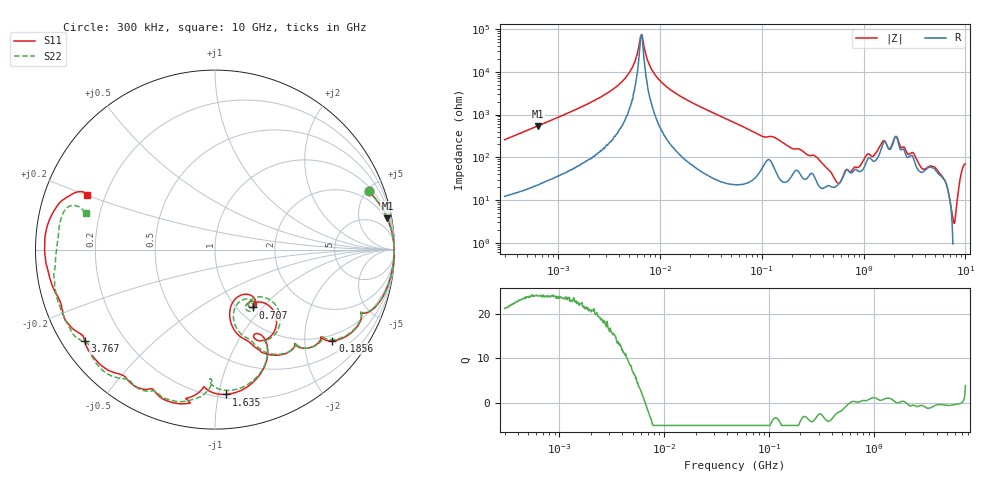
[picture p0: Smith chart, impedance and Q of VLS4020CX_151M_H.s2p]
! S-Parameter Data Generated by TDK Corporation
! Copyright(C) 2024 TDK Corporation.
! All Rights Reserved.
! TDK P/N: VLS4020CX-151M-H (SMD / SMT Inductor (Coil))
! Property: L=150uH at 1MHz
! Size(LxWxT): 4x4x2mm
! Model Type: s2p (Touchstone File Format Version 1.0)
! Frequency: DC=Yes Start=0.3MHz Stop=10000MHz 802points Log-sweep
! Model Generated on May 28, 2024
! Terms and conditions regarding TDK Simulation Models:
! 1)This simulation model is being provided solely for informational
!  purposes. Please refer to the specifications of the products in
!  terms of detailed characteristics of such products.
! 2)In no event shall TDK Corporation of any of its subsidiaries be
!  liable for any loss or damage arising, directly or indirectly,
!  from any information contained in this simulation model, including,
!  but not limited to loss or damages arising from any inaccuracies,
!  omissions or errors in connection with such information.
! 3)Any and all copyrights on this simulation model are owned by
!  TDK Corporation.  Duplication or redistribution of this simulation
!  model without prior written permission from TDK Corporation
!  is prohibited.
! 4)This simulation model is subject to any modification or change
!  without any prior notice.
! 5)Neither TDK Corporation nor any of its subsidiaries shall make any
!  warranty, express or implied, including but not limited to the
!  correctness, implied warranties of merchantability and fitness for
!  a particular purpose with respect to this simulation models.
! 6)The use of this simulation model shall be deemed to have consented
!  to the terms and conditions hereof.
! Port Assignments:
!  1 ---@@@--- 2
! Applicable Conditions:
!  Temperature = 25 degC
!  DC Bias Current = 0 A
!  Small Signal Operation
# Hz S MA R 50
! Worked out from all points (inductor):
!   801 points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, 300 kHz to 10 GHz, reference 50 ohm
!   read as one part in series: L = 135 uH near 318.3 kHz
!   highest Q = 24 at 636.7 kHz (marker M1), where L = 135 uH
!   self-resonance near 6.556 MHz
!   S11 on the Smith chart (normalised r, x): 300 kHz: 1.27, +5.17; 185.6 MHz: 0.83, -2.69; 707 MHz: 1.17, -0.89; 1.635 GHz: 0.23, -1.05; 3.767 GHz: 0.07, -0.31; 10 GHz: 0.13, +0.20
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300000  0.9171 20.7  0.3572 -66.6  0.3572 -66.6  0.9173 20.7
636701  0.9761 10.3  0.1803 -77.3  0.1802 -77.3  0.976 10.3
1713600  0.9949 3.6  0.0656 -83.7  0.06573 -83.7  0.9948 3.6
4487199  0.9984 0.5  0.01487 -83.6  0.01488 -83.5  0.9983 0.5
5416338  0.9986 0.1  0.007638 -80.1  0.007654 -79.6  0.9987 0.1
6556275  0.9987 -0.4  0.001397 -14.9  0.00132 -12.1  0.9987 -0.4
7771787  0.9987 -0.9  0.00614 77.4  0.006137 77.1  0.9988 -0.8
9671944  0.9985 -1.5  0.01459 83.5  0.01462 83.5  0.9987 -1.5
5.477226e7  0.9828 -12.3  0.1533 75.7  0.1534 75.7  0.9827 -12.2
1.855783e8  0.8285 -37.9  0.441 43.4  0.4411 43.4  0.8312 -37.1
3.126428e8  0.691 -49.9  0.5286 21.1  0.5287 21.1  0.6903 -49.3
5.225392e8  0.4301 -77.5  0.7491 -7.9  0.7493 -7.9  0.4364 -75.1
7.069847e8  0.3847 -56.9  0.6277 -32.2  0.6278 -32.2  0.3959 -60.3
9.789263e8  0.4268 -46.2  0.5948 -64.1  0.5949 -64.2  0.3845 -43.9
1.371335e9  0.6406 -62.7  0.3677 -94.6  0.3679 -94.6  0.6674 -64.3
1.635219e9  0.8091 -85.6  0.1862 -83.5  0.1864 -83.5  0.7835 -86.8
1.767019e9  0.7729 -94.0  0.2329 -82.6  0.233 -82.7  0.7231 -92.4
2.112126e9  0.8836 -104.2  0.1123 -80.9  0.1124 -80.9  0.8677 -102.4
3.766866e9  0.8875 -145.0  0.162 -85.5  0.1619 -85.7  0.8922 -141.6
5.849356e9  0.9105 -160.4  0.09971 -108.6  0.09939 -108.7  0.9218 -153.8
7.540283e9  0.9495 180.0  0.07683 -126.5  0.0769 -126.5  0.8913 -175.6
1e10  0.7749 156.7  0.05116 -125.5  0.05123 -125.6  0.7493 164.3
